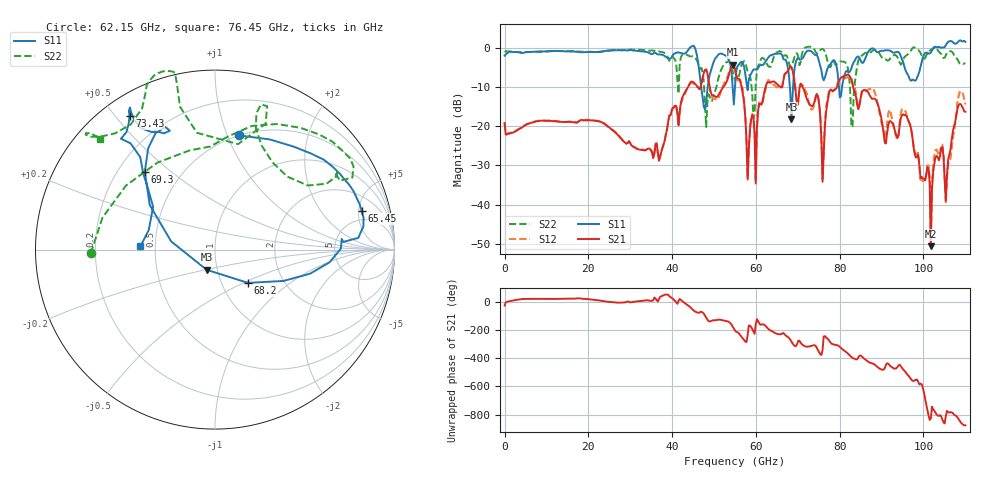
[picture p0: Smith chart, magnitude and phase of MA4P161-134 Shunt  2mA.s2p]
!Keysight Technologies,N5247B,US61255204,A.15.70.20
!Date: Friday, October 21, 2022 14:11:56
!Correction: S11(C  4-Port  )
!S31(C  4-Port  )
!S13(C  4-Port  )
!S33(C  4-Port  )
!S2P File: Measurements: S11, S31, S13, S33:
# Hz S  dB  R 50
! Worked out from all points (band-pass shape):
!   401 points, 10 MHz to 110 GHz, reference 50 ohm
!   highest |S21| = -4.29 dB at 54.46 GHz (marker M1); lowest = -50.6 dB at 101.8 GHz (marker M2)
!   |S21| within 3 dB of the highest: 53.46 GHz to 55.44 GHz (1.984 GHz wide, 3.64 % of centre); 66.74 GHz to 69.04 GHz (2.292 GHz wide, 3.38 % of centre)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
!   lowest |S11| = -18.3 dB at 68.48 GHz (marker M3), VSWR 1.28, Z = 44.5 - j10.2 ohm
!   |S11| at or under -10 dB: 46.93 GHz to 48.5 GHz (1.569 GHz wide, 3.29 % of centre); 54.45 GHz to 55 GHz (554.1 MHz wide, 1.01 % of centre); 68.09 GHz to 68.87 GHz (776.3 MHz wide, 1.13 % of centre)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
!   |S22| runs from -20.3 to 0.3 dB; largest |S21 - S12| = 0.16
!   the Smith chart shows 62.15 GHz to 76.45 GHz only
!   S11 on the Smith chart (normalised r, x): 62.15 GHz: 0.50, +1.10; 65.45 GHz: 3.59, +5.40; 68.2 GHz: 1.33, -0.53; 69.3 GHz: 0.31, +0.41; 73.43 GHz: 0.08, +0.55; 76.45 GHz: 0.41, +0.02
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1e7  -2.00 -176.9  -19.18 -24.0  -19.16 -23.9  -1.07 -177.0
1.843332e10  -1.11 130.7  -18.42 24.6  -18.43 24.6  -0.97 140.5
3.685665e10  -1.66 126.3  -28.84 22.7  -28.69 22.9  -0.92 133.7
4.565585e10  -0.70 52.4  -9.40 -68.8  -9.77 -67.1  -2.78 27.1
5.445505e10  -10.09 98.3  -4.29 -174.1  -4.36 -173.8  -5.96 127.5
5.5005e10  -9.97 -177.6  -5.34 158.7  -5.55 158.4  -8.30 148.0
5.802972e10  -10.84 159.3  -33.63 127.7  -33.32 127.5  -6.14 167.5
6.077948e10  -4.70 149.6  -14.31 -149.4  -13.96 -150.3  -4.15 -121.9
6.215435e10  -3.74 78.0  -10.51 -165.0  -11.22 -159.3  -3.19 -178.3
6.545405e10  -1.46 14.7  -9.68 132.0  -9.70 154.0  -0.93 37.9
6.82038e10  -11.66 -45.2  -4.75 93.0  -4.91 90.3  -4.85 45.3
6.847878e10  -18.29 -112.5  -4.92 79.6  -5.12 77.5  -4.70 56.6
6.93037e10  -4.67 132.0  -9.47 47.7  -9.22 47.2  -2.01 73.1
7.342832e10  -1.06 122.6  -14.90 51.0  -15.76 49.4  0.10 111.0
7.645305e10  -7.62 177.5  -20.34 118.5  -19.36 130.7  -1.01 136.0
8.085265e10  -8.15 -75.9  -7.25 20.5  -7.68 21.1  -3.51 -144.0
8.305245e10  -4.35 -45.6  -9.31 -37.0  -8.78 -20.6  -20.29 10.9
8.607718e10  -2.78 6.3  -10.87 -47.4  -10.72 -46.0  -1.28 -14.8
9.185165e10  -0.67 71.6  -18.76 -86.0  -15.80 -82.9  -3.02 67.1
9.762612e10  -8.18 177.7  -25.37 158.7  -24.86 156.8  0.14 166.0
1.017508e11  -1.16 -88.2  -50.63 -108.1  -48.58 -91.2  -0.49 -124.6
1.1e11  1.53 8.3  -16.32 -156.7  -14.44 -161.4  -4.04 16.6
